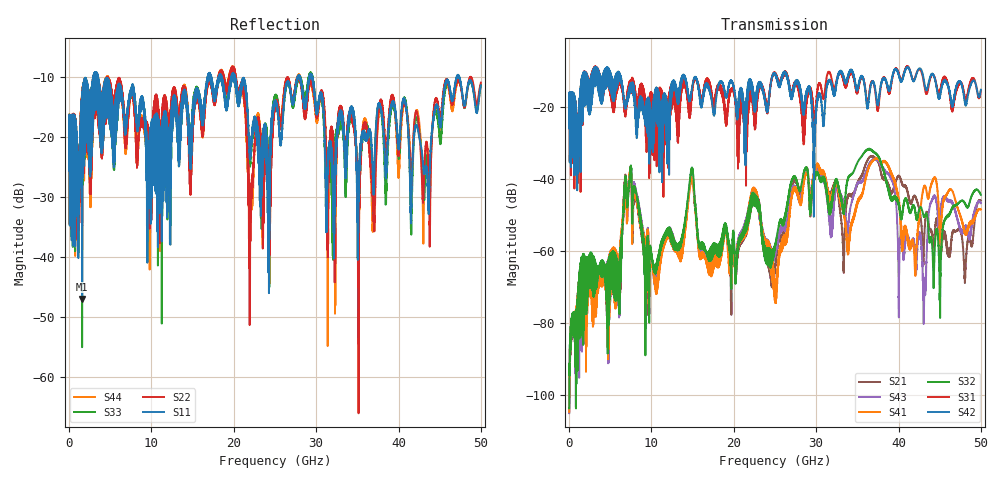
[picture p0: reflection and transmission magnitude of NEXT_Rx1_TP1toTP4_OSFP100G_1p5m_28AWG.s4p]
! Touchstone data
! Created: 27-Feb-2019 by IdEM 12 (12.1.0)
! COMMENTS
!  Created Wed Feb 27 09:43:39 2019
!  64 Port Network Data from SP1.SP block
!  freq  magS1_1  angS1_1  magS1_2  angS1_2  magS1_3  angS1_3  magS1_4  angS1_4
!  magS1_5  angS1_5  magS1_6  angS1_6  magS1_7  angS1_7  magS1_8  angS1_8
!  magS1_9  angS1_9  magS1_10  angS1_10  magS1_11  angS1_11  magS1_12  angS1_12
!  magS1_13  angS1_13  magS1_14  angS1_14  magS1_15  angS1_15  magS1_16  angS1_16
!  magS1_17  angS1_17  magS1_18  angS1_18  magS1_19  angS1_19  magS1_20  angS1_20
!  magS1_21  angS1_21  magS1_22  angS1_22  magS1_23  angS1_23  magS1_24  angS1_24
!  magS1_25  angS1_25  magS1_26  angS1_26  magS1_27  angS1_27  magS1_28  angS1_28
!  magS1_29  angS1_29  magS1_30  angS1_30  magS1_31  angS1_31  magS1_32  angS1_32
!  magS1_33  angS1_33  magS1_34  angS1_34  magS1_35  angS1_35  magS1_36  angS1_36
!  magS1_37  angS1_37  magS1_38  angS1_38  magS1_39  angS1_39  magS1_40  angS1_40
!  magS1_41  angS1_41  magS1_42  angS1_42  magS1_43  angS1_43  magS1_44  angS1_44
!  magS1_45  angS1_45  magS1_46  angS1_46  magS1_47  angS1_47  magS1_48  angS1_48
!  magS1_49  angS1_49  magS1_50  angS1_50  magS1_51  angS1_51  magS1_52  angS1_52
!  magS1_53  angS1_53  magS1_54  angS1_54  magS1_55  angS1_55  magS1_56  angS1_56
!  magS1_57  angS1_57  magS1_58  angS1_58  magS1_59  angS1_59  magS1_60  angS1_60
!  magS1_61  angS1_61  magS1_62  angS1_62  magS1_63  angS1_63  magS1_64  angS1_64
!  magS2_1  angS2_1  magS2_2  angS2_2  magS2_3  angS2_3  magS2_4  angS2_4
!  magS2_5  angS2_5  magS2_6  angS2_6  magS2_7  angS2_7  magS2_8  angS2_8
!  magS2_9  angS2_9  magS2_10  angS2_10  magS2_11  angS2_11  magS2_12  angS2_12
!  magS2_13  angS2_13  magS2_14  angS2_14  magS2_15  angS2_15  magS2_16  angS2_16
!  magS2_17  angS2_17  magS2_18  angS2_18  magS2_19  angS2_19  magS2_20  angS2_20
!  magS2_21  angS2_21  magS2_22  angS2_22  magS2_23  angS2_23  magS2_24  angS2_24
!  magS2_25  angS2_25  magS2_26  angS2_26  magS2_27  angS2_27  magS2_28  angS2_28
!  magS2_29  angS2_29  magS2_30  angS2_30  magS2_31  angS2_31  magS2_32  angS2_32
!  magS2_33  angS2_33  magS2_34  angS2_34  magS2_35  angS2_35  magS2_36  angS2_36
!  magS2_37  angS2_37  magS2_38  angS2_38  magS2_39  angS2_39  magS2_40  angS2_40
!  magS2_41  angS2_41  magS2_42  angS2_42  magS2_43  angS2_43  magS2_44  angS2_44
!  magS2_45  angS2_45  magS2_46  angS2_46  magS2_47  angS2_47  magS2_48  angS2_48
!  magS2_49  angS2_49  magS2_50  angS2_50  magS2_51  angS2_51  magS2_52  angS2_52
!  magS2_53  angS2_53  magS2_54  angS2_54  magS2_55  angS2_55  magS2_56  angS2_56
!  magS2_57  angS2_57  magS2_58  angS2_58  magS2_59  angS2_59  magS2_60  angS2_60
!  magS2_61  angS2_61  magS2_62  angS2_62  magS2_63  angS2_63  magS2_64  angS2_64
!  magS3_1  angS3_1  magS3_2  angS3_2  magS3_3  angS3_3  magS3_4  angS3_4
!  magS3_5  angS3_5  magS3_6  angS3_6  magS3_7  angS3_7  magS3_8  angS3_8
!  magS3_9  angS3_9  magS3_10  angS3_10  magS3_11  angS3_11  magS3_12  angS3_12
!  magS3_13  angS3_13  magS3_14  angS3_14  magS3_15  angS3_15  magS3_16  angS3_16
!  magS3_17  angS3_17  magS3_18  angS3_18  magS3_19  angS3_19  magS3_20  angS3_20
!  magS3_21  angS3_21  magS3_22  angS3_22  magS3_23  angS3_23  magS3_24  angS3_24
!  magS3_25  angS3_25  magS3_26  angS3_26  magS3_27  angS3_27  magS3_28  angS3_28
!  magS3_29  angS3_29  magS3_30  angS3_30  magS3_31  angS3_31  magS3_32  angS3_32
!  magS3_33  angS3_33  magS3_34  angS3_34  magS3_35  angS3_35  magS3_36  angS3_36
!  magS3_37  angS3_37  magS3_38  angS3_38  magS3_39  angS3_39  magS3_40  angS3_40
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# Hz S MA R 50
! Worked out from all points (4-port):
!   5000 points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, 10 MHz to 50 GHz, reference 50 ohm
!   strongest paths, dB at 10 MHz, 12.51 GHz, 25.01 GHz, 37.51 GHz, 50 GHz:
!     S42: -19.6, -13.3, -11.0, -19.1, -15.1
!     S31: -19.6, -16.2, -10.8, -21.0, -15.4
!     S32: -103.6, -57.4, -59.2, -33.6, -44.3
!     S41: -104.6, -57.7, -69.9, -34.3, -48.4
!     S43: -104.9, -56.8, -60.5, -34.9, -46.6
!     S21: -104.6, -58.0, -65.1, -35.2, -46.0
!   lowest |S11| = -47.1 dB at 1.59 GHz (marker M1), VSWR 1.01, Z = 49.7 + j0.298 ohm
!   |S11| at or under -10 dB: 3.482 GHz to 16.85 GHz (13.37 GHz wide, 132 % of centre); 20.15 GHz to 27.79 GHz (7.635 GHz wide, 31.9 % of centre); 29.53 GHz to 47.08 GHz (17.55 GHz wide, 45.8 % of centre)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
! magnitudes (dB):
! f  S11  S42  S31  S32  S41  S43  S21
! 10 MHz  -19.2  -19.6  -19.6  -103.6  -104.6  -104.9  -104.6
! 1.59 GHz  -47.1  -24.7  -24.2  -62.1  -62.2  -62.2  -62.4
! 7.4 GHz  -12.5  -14.0  -13.2  -38.3  -38.0  -38.3  -38.1
! 10.57 GHz  -16.3  -14.6  -18.4  -65.4  -70.6  -69.9  -66.7
! 14.89 GHz  -18.4  -15.2  -16.2  -36.8  -39.5  -38.0  -38.2
! 25.02 GHz  -14.2  -10.9  -11.0  -58.5  -73.5  -61.0  -64.4
! 50 GHz  -11.5  -15.1  -15.4  -44.3  -48.4  -46.6  -46.0
